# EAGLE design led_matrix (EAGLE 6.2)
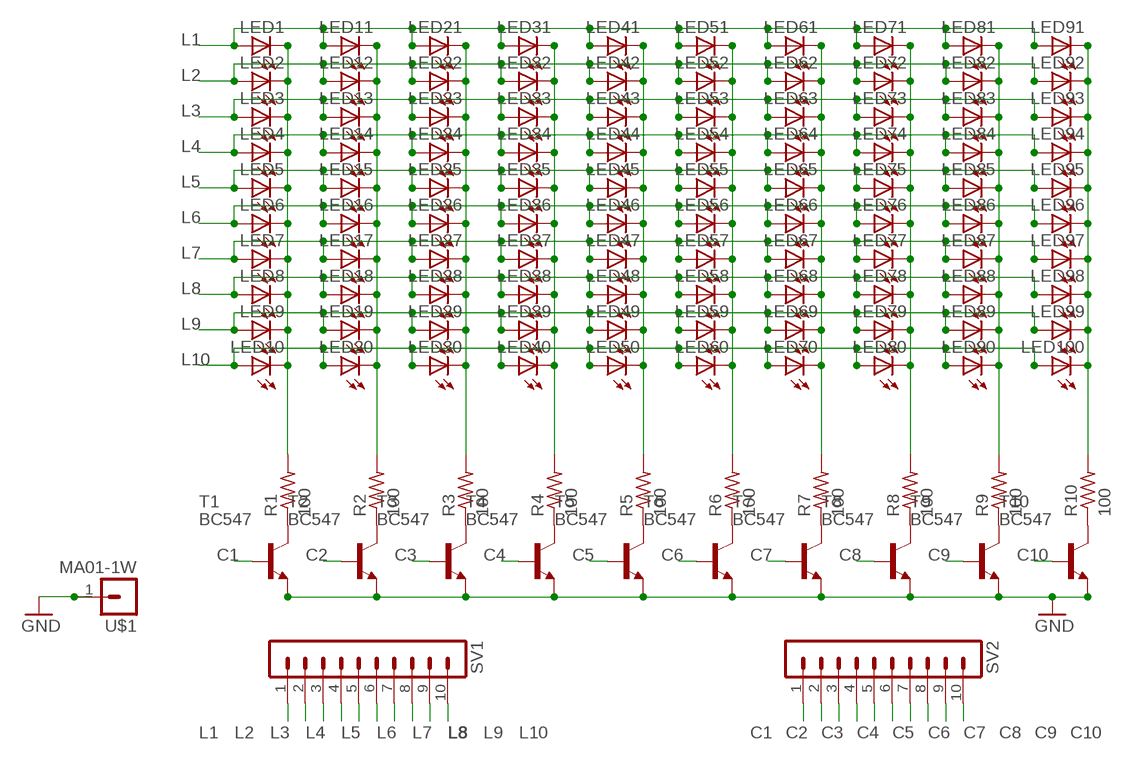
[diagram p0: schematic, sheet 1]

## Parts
LED1  LED5MM  [LED5MM]
LED2  LED5MM  [LED5MM]
LED3  LED5MM  [LED5MM]
LED4  LED5MM  [LED5MM]
LED5  LED5MM  [LED5MM]
LED6  LED5MM  [LED5MM]
LED7  LED5MM  [LED5MM]
LED8  LED5MM  [LED5MM]
LED9  LED5MM  [LED5MM]
LED10  LED5MM  [LED5MM]
LED11  LED5MM  [LED5MM]
LED12  LED5MM  [LED5MM]
LED13  LED5MM  [LED5MM]
LED14  LED5MM  [LED5MM]
LED15  LED5MM  [LED5MM]
LED16  LED5MM  [LED5MM]
LED17  LED5MM  [LED5MM]
LED18  LED5MM  [LED5MM]
LED19  LED5MM  [LED5MM]
LED20  LED5MM  [LED5MM]
LED21  LED5MM  [LED5MM]
LED22  LED5MM  [LED5MM]
LED23  LED5MM  [LED5MM]
LED24  LED5MM  [LED5MM]
LED25  LED5MM  [LED5MM]
LED26  LED5MM  [LED5MM]
LED27  LED5MM  [LED5MM]
LED28  LED5MM  [LED5MM]
LED29  LED5MM  [LED5MM]
LED30  LED5MM  [LED5MM]
LED31  LED5MM  [LED5MM]
LED32  LED5MM  [LED5MM]
LED33  LED5MM  [LED5MM]
LED34  LED5MM  [LED5MM]
LED35  LED5MM  [LED5MM]
LED36  LED5MM  [LED5MM]
LED37  LED5MM  [LED5MM]
LED38  LED5MM  [LED5MM]
LED39  LED5MM  [LED5MM]
LED40  LED5MM  [LED5MM]
LED41  LED5MM  [LED5MM]
LED42  LED5MM  [LED5MM]
LED43  LED5MM  [LED5MM]
LED44  LED5MM  [LED5MM]
LED45  LED5MM  [LED5MM]
LED46  LED5MM  [LED5MM]
LED47  LED5MM  [LED5MM]
LED48  LED5MM  [LED5MM]
LED49  LED5MM  [LED5MM]
LED50  LED5MM  [LED5MM]
LED51  LED5MM  [LED5MM]
LED52  LED5MM  [LED5MM]
LED53  LED5MM  [LED5MM]
LED54  LED5MM  [LED5MM]
LED55  LED5MM  [LED5MM]
LED56  LED5MM  [LED5MM]
LED57  LED5MM  [LED5MM]
LED58  LED5MM  [LED5MM]
LED59  LED5MM  [LED5MM]
LED60  LED5MM  [LED5MM]
LED61  LED5MM  [LED5MM]
LED62  LED5MM  [LED5MM]
LED63  LED5MM  [LED5MM]
LED64  LED5MM  [LED5MM]
LED65  LED5MM  [LED5MM]
LED66  LED5MM  [LED5MM]
LED67  LED5MM  [LED5MM]
LED68  LED5MM  [LED5MM]
LED69  LED5MM  [LED5MM]
LED70  LED5MM  [LED5MM]
LED71  LED5MM  [LED5MM]
LED72  LED5MM  [LED5MM]
LED73  LED5MM  [LED5MM]
LED74  LED5MM  [LED5MM]
LED75  LED5MM  [LED5MM]
LED76  LED5MM  [LED5MM]
LED77  LED5MM  [LED5MM]
LED78  LED5MM  [LED5MM]
LED79  LED5MM  [LED5MM]
LED80  LED5MM  [LED5MM]
LED81  LED5MM  [LED5MM]
LED82  LED5MM  [LED5MM]
LED83  LED5MM  [LED5MM]
LED84  LED5MM  [LED5MM]
LED85  LED5MM  [LED5MM]
LED86  LED5MM  [LED5MM]
LED87  LED5MM  [LED5MM]
LED88  LED5MM  [LED5MM]
LED89  LED5MM  [LED5MM]
LED90  LED5MM  [LED5MM]
LED91  LED5MM  [LED5MM]
LED92  LED5MM  [LED5MM]
LED93  LED5MM  [LED5MM]
LED94  LED5MM  [LED5MM]
LED95  LED5MM  [LED5MM]
LED96  LED5MM  [LED5MM]
LED97  LED5MM  [LED5MM]
LED98  LED5MM  [LED5MM]
LED99  LED5MM  [LED5MM]
LED100  LED5MM  [LED5MM]
R1  100  R-US_0207/10  [0207/10]
R2  100  R-US_0207/10  [0207/10]
R3  100  R-US_0207/10  [0207/10]
R4  100  R-US_0207/10  [0207/10]
R5  100  R-US_0207/10  [0207/10]
R6  100  R-US_0207/10  [0207/10]
R7  100  R-US_0207/10  [0207/10]
R8  100  R-US_0207/10  [0207/10]
R9  100  R-US_0207/10  [0207/10]
R10  100  R-US_0207/10  [0207/10]
SV1  MA10-1W  [MA10-1W]
SV2  MA10-1W  [MA10-1W]
T1  BC547  BC618  [TO92-EBC]
T2  BC547  BC618  [TO92-EBC]
T3  BC547  BC618  [TO92-EBC]
T4  BC547  BC618  [TO92-EBC]
T5  BC547  BC618  [TO92-EBC]
T6  BC547  BC618  [TO92-EBC]
T7  BC547  BC618  [TO92-EBC]
T8  BC547  BC618  [TO92-EBC]
T9  BC547  BC618  [TO92-EBC]
T10  BC547  BC618  [TO92-EBC]
U$1  MA01-1W  [MA01-1W]

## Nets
C1: SV2.1 T1.B
C2: SV2.2 T2.B
C3: SV2.3 T3.B
C4: SV2.4 T4.B
C5: SV2.5 T5.B
C6: SV2.6 T6.B
C7: SV2.7 T7.B
C8: SV2.8 T8.B
C9: SV2.9 T9.B
C10: SV2.10 T10.B
GND: T1.E T2.E T3.E T4.E T5.E T6.E T7.E T8.E T9.E T10.E U$1.1
L1: LED1.A LED11.A LED21.A LED31.A LED41.A LED51.A LED61.A LED71.A LED81.A LED91.A SV1.1
L2: LED2.A LED12.A LED22.A LED32.A LED42.A LED52.A LED62.A LED72.A LED82.A LED92.A SV1.2
L3: LED3.A LED13.A LED23.A LED33.A LED43.A LED53.A LED63.A LED73.A LED83.A LED93.A SV1.3
L4: LED4.A LED14.A LED24.A LED34.A LED44.A LED54.A LED64.A LED74.A LED84.A LED94.A SV1.4
L5: LED5.A LED15.A LED25.A LED35.A LED45.A LED55.A LED65.A LED75.A LED85.A LED95.A SV1.5
L6: LED6.A LED16.A LED26.A LED36.A LED46.A LED56.A LED66.A LED76.A LED86.A LED96.A SV1.6
L7: LED7.A LED17.A LED27.A LED37.A LED47.A LED57.A LED67.A LED77.A LED87.A LED97.A SV1.7
L8: LED8.A LED18.A LED28.A LED38.A LED48.A LED58.A LED68.A LED78.A LED88.A LED98.A SV1.8
L9: LED9.A LED19.A LED29.A LED39.A LED49.A LED59.A LED69.A LED79.A LED89.A LED99.A SV1.9
L10: LED10.A LED20.A LED30.A LED40.A LED50.A LED60.A LED70.A LED80.A LED90.A LED100.A SV1.10
N$1: R1.1 T1.C
N$2: R2.1 T2.C
N$3: R3.1 T3.C
N$4: R4.1 T4.C
N$5: R5.1 T5.C
N$6: R6.1 T6.C
N$7: R7.1 T7.C
N$8: R8.1 T8.C
N$9: R9.1 T9.C
N$10: R10.1 T10.C
N$11: LED1.K(C) LED2.K(C) LED3.K(C) LED4.K(C) LED5.K(C) LED6.K(C) LED7.K(C) LED8.K(C) LED9.K(C) LED10.K(C) R1.2
N$12: LED11.K(C) LED12.K(C) LED13.K(C) LED14.K(C) LED15.K(C) LED16.K(C) LED17.K(C) LED18.K(C) LED19.K(C) LED20.K(C) R2.2
N$13: LED21.K(C) LED22.K(C) LED23.K(C) LED24.K(C) LED25.K(C) LED26.K(C) LED27.K(C) LED28.K(C) LED29.K(C) LED30.K(C) R3.2
N$14: LED31.K(C) LED32.K(C) LED33.K(C) LED34.K(C) LED35.K(C) LED36.K(C) LED37.K(C) LED38.K(C) LED39.K(C) LED40.K(C) R4.2
N$15: LED41.K(C) LED42.K(C) LED43.K(C) LED44.K(C) LED45.K(C) LED46.K(C) LED47.K(C) LED48.K(C) LED49.K(C) LED50.K(C) R5.2
N$16: LED51.K(C) LED52.K(C) LED53.K(C) LED54.K(C) LED55.K(C) LED56.K(C) LED57.K(C) LED58.K(C) LED59.K(C) LED60.K(C) R6.2
N$17: LED61.K(C) LED62.K(C) LED63.K(C) LED64.K(C) LED65.K(C) LED66.K(C) LED67.K(C) LED68.K(C) LED69.K(C) LED70.K(C) R7.2
N$18: LED71.K(C) LED72.K(C) LED73.K(C) LED74.K(C) LED75.K(C) LED76.K(C) LED77.K(C) LED78.K(C) LED79.K(C) LED80.K(C) R8.2
N$19: LED81.K(C) LED82.K(C) LED83.K(C) LED84.K(C) LED85.K(C) LED86.K(C) LED87.K(C) LED88.K(C) LED89.K(C) LED90.K(C) R9.2
N$20: LED91.K(C) LED92.K(C) LED93.K(C) LED94.K(C) LED95.K(C) LED96.K(C) LED97.K(C) LED98.K(C) LED99.K(C) LED100.K(C) R10.2

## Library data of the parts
LED1-LED100 = SparkFun-LED:LED: LEDs
R1-R10 = rcl:R-US_: RESISTOR, American symbol
SV1 SV2 = con-lstb:MA10-1W: PIN HEADER; OC_FARNELL: unknown; OC_NEWARK: unknown
T1-T10 = transistor-npn:BC618*: NPN Transistor
U$1 = con-lstb:MA01-1W

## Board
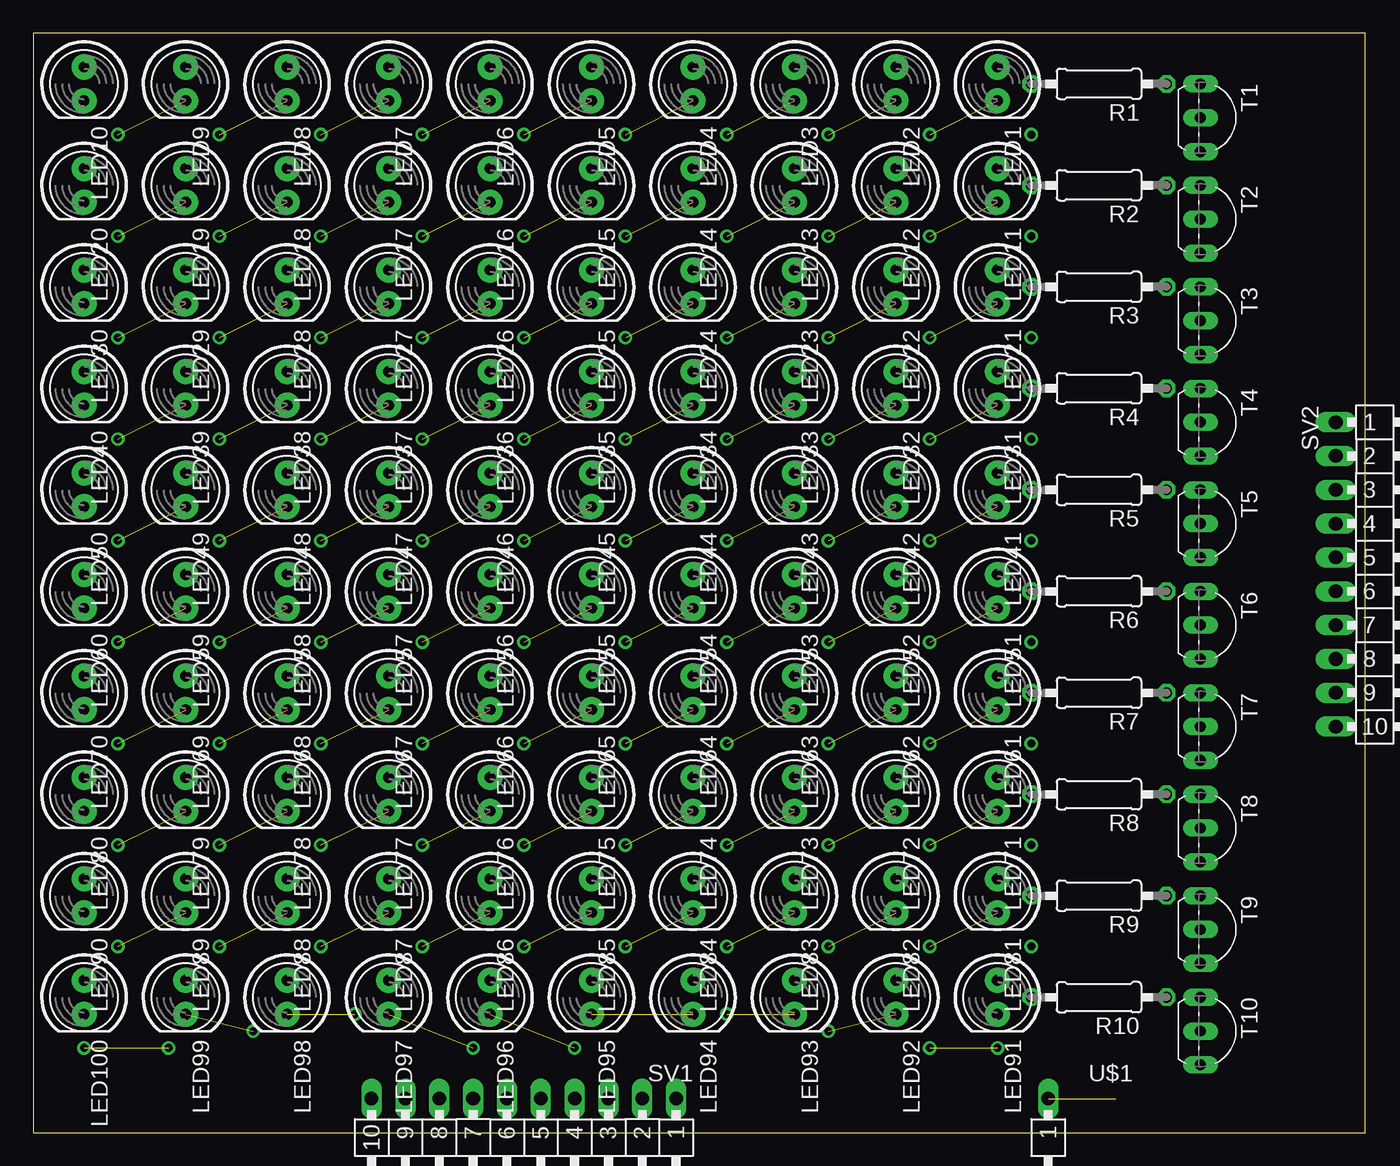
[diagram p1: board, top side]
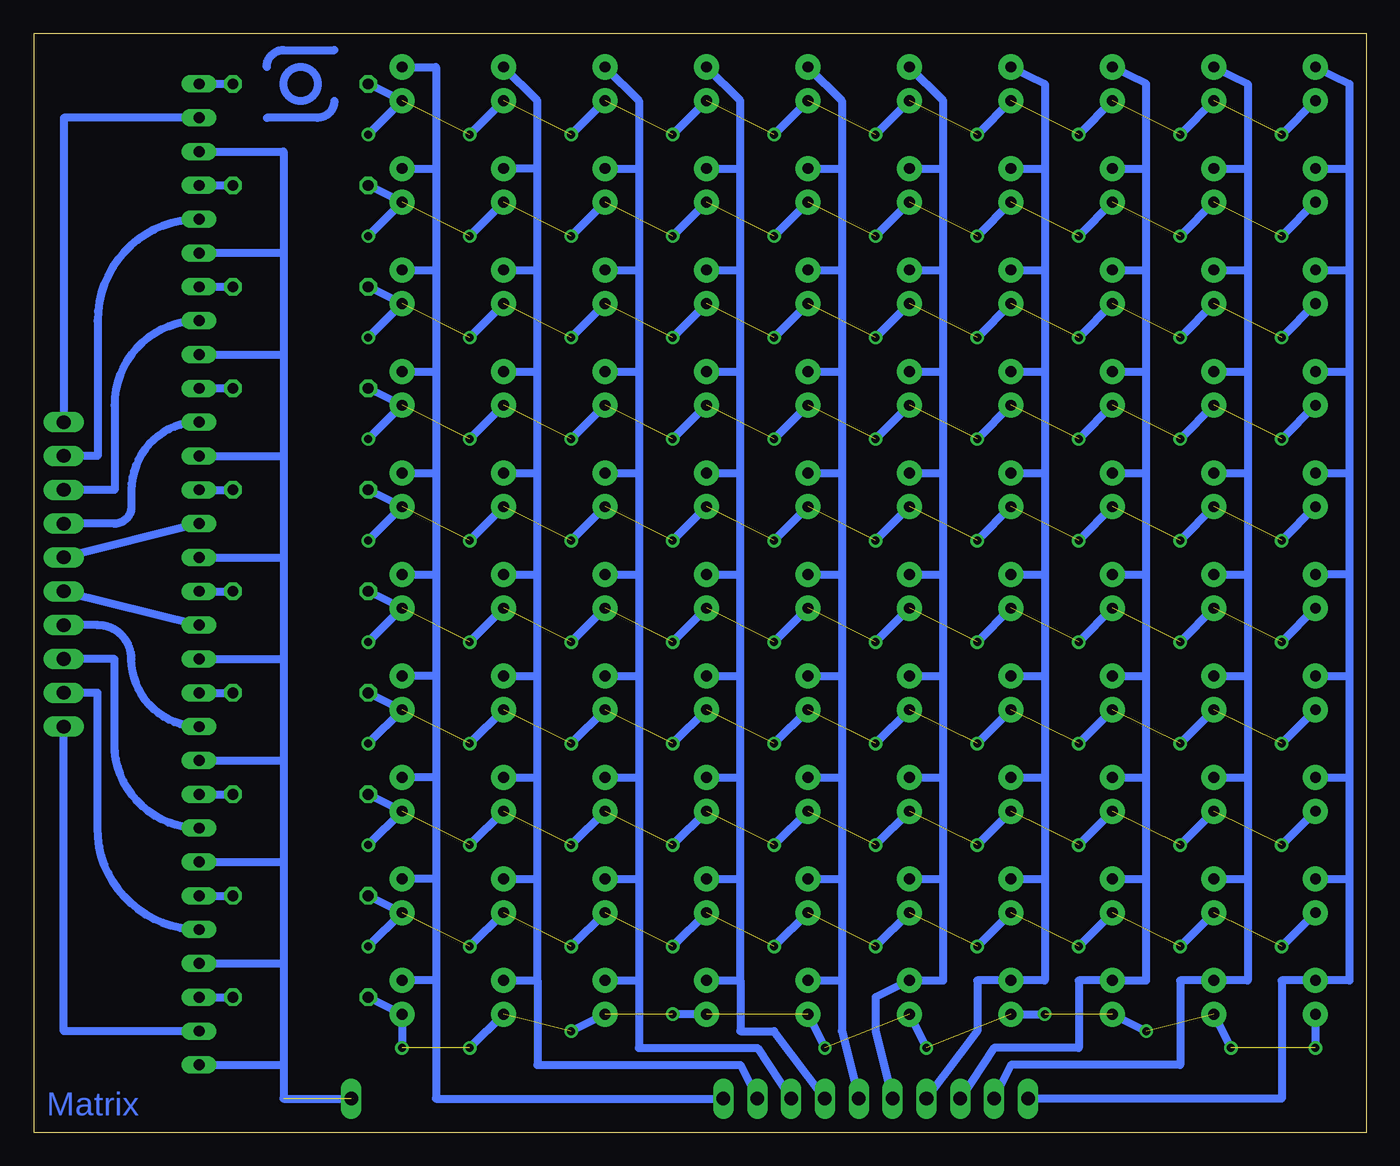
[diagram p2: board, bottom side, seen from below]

Size 100 x 82.54 mm. Coordinates in mm from the lower left corner, seen from the top.
Outline: 0,0 100,0 100,82.54 0,82.54 0,0
Copper layers (1*16): Top 0.035mm / dielectric 1.5mm / Bottom 0.035mm
Design rules: minimum track width 0.5mm, minimum drill 0.6mm, track to track 0.5mm, track to pad 0.5mm, pad to pad 0.5mm, via to via 0.5mm, smd to smd 8mil, copper to edge 0.4mm, drill to drill 8mil, minimum pad ring 10mil, minimum via ring 8mil, stop-mask expansion 4mil, vias tented up to drill 0mil, thermal gap 10mil

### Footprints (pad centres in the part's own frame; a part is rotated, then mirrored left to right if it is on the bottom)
LED5MM = drill 0.813 pad 1.88: A -1.27,0; K 1.27,0
0207/10 = drill 0.813 octagon: 1 -5.08,0; 2 5.08,0
MA10-1W = drill 1.016 long: 1 -11.43,0; 2 -8.89,0; 3 -6.35,0; 4 -3.81,0; 5 -1.27,0; 6 1.27,0; 7 3.81,0; 8 6.35,0; 9 8.89,0; 10 11.43,0
TO92-EBC = drill 0.813 long: B 0,-1.27; C -2.54,-1.27; E 2.54,-1.27
MA01-1W = drill 1.016 long: 1 6.35,2.54

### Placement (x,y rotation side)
LED1  72.39,78.74 270 top
LED2  64.77,78.74 270 top
LED3  57.15,78.74 270 top
LED4  49.53,78.74 270 top
LED5  41.91,78.74 270 top
LED6  34.29,78.74 270 top
LED7  26.67,78.74 270 top
LED8  19.05,78.74 270 top
LED9  11.43,78.74 270 top
LED10  3.81,78.74 270 top
LED11  72.39,71.12 270 top
LED12  64.77,71.12 270 top
LED13  57.15,71.12 270 top
LED14  49.53,71.12 270 top
LED15  41.91,71.12 270 top
LED16  34.29,71.12 270 top
LED17  26.67,71.12 270 top
LED18  19.05,71.12 270 top
LED19  11.43,71.12 270 top
LED20  3.81,71.12 270 top
LED21  72.39,63.5 270 top
LED22  64.77,63.5 270 top
LED23  57.15,63.5 270 top
LED24  49.53,63.5 270 top
LED25  41.91,63.5 270 top
LED26  34.29,63.5 270 top
LED27  26.67,63.5 270 top
LED28  19.05,63.5 270 top
LED29  11.43,63.5 270 top
LED30  3.81,63.5 270 top
LED31  72.39,55.88 270 top
LED32  64.77,55.88 270 top
LED33  57.15,55.88 270 top
LED34  49.53,55.88 270 top
LED35  41.91,55.88 270 top
LED36  34.29,55.88 270 top
LED37  26.67,55.88 270 top
LED38  19.05,55.88 270 top
LED39  11.43,55.88 270 top
LED40  3.81,55.88 270 top
LED41  72.39,48.26 270 top
LED42  64.77,48.26 270 top
LED43  57.15,48.26 270 top
LED44  49.53,48.26 270 top
LED45  41.91,48.26 270 top
LED46  34.29,48.26 270 top
LED47  26.67,48.26 270 top
LED48  19.05,48.26 270 top
LED49  11.43,48.26 270 top
LED50  3.81,48.26 270 top
LED51  72.39,40.64 270 top
LED52  64.77,40.64 270 top
LED53  57.15,40.64 270 top
LED54  49.53,40.64 270 top
LED55  41.91,40.64 270 top
LED56  34.29,40.64 270 top
LED57  26.67,40.64 270 top
LED58  19.05,40.64 270 top
LED59  11.43,40.64 270 top
LED60  3.81,40.64 270 top
LED61  72.39,33.02 270 top
LED62  64.77,33.02 270 top
LED63  57.15,33.02 270 top
LED64  49.53,33.02 270 top
LED65  41.91,33.02 270 top
LED66  34.29,33.02 270 top
LED67  26.67,33.02 270 top
LED68  19.05,33.02 270 top
LED69  11.43,33.02 270 top
LED70  3.81,33.02 270 top
LED71  72.39,25.4 270 top
LED72  64.77,25.4 270 top
LED73  57.15,25.4 270 top
LED74  49.53,25.4 270 top
LED75  41.91,25.4 270 top
LED76  34.29,25.4 270 top
LED77  26.67,25.4 270 top
LED78  19.05,25.4 270 top
LED79  11.43,25.4 270 top
LED80  3.81,25.4 270 top
LED81  72.39,17.78 270 top
LED82  64.77,17.78 270 top
LED83  57.15,17.78 270 top
LED84  49.53,17.78 270 top
LED85  41.91,17.78 270 top
LED86  34.29,17.78 270 top
LED87  26.67,17.78 270 top
LED88  19.05,17.78 270 top
LED89  11.43,17.78 270 top
LED90  3.81,17.78 270 top
LED91  72.39,10.16 270 top
LED92  64.77,10.16 270 top
LED93  57.15,10.16 270 top
LED94  49.53,10.16 270 top
LED95  41.91,10.16 270 top
LED96  34.29,10.16 270 top
LED97  26.67,10.16 270 top
LED98  19.05,10.16 270 top
LED99  11.43,10.16 270 top
LED100  3.81,10.16 270 top
R1  80.01,78.74 180 top
R2  80.01,71.12 180 top
R3  80.01,63.5 180 top
R4  80.01,55.88 180 top
R5  80.01,48.26 180 top
R6  80.01,40.64 180 top
R7  80.01,33.02 180 top
R8  80.01,25.4 180 top
R9  80.01,17.78 180 top
R10  80.01,10.16 180 top
SV1  36.83,2.54 180 top
SV2  97.79,41.91 270 top
T1  88.9,76.2 270 top
T2  88.9,68.58 270 top
T3  88.9,60.96 270 top
T4  88.9,53.34 270 top
T5  88.9,45.72 270 top
T6  88.9,38.1 270 top
T7  88.9,30.48 270 top
T8  88.9,22.86 270 top
T9  88.9,15.24 270 top
T10  88.9,7.62 270 top
U$1  82.55,5.08 180 top

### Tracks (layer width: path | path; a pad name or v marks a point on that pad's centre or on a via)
C1
  Bottom 0.6: T1.B 97.79,76.2 SV2.1
C2
  Bottom 0.6: T2.B arc-90 95.25,60.96 95.25,50.8 SV2.2
C3
  Bottom 0.6: T3.B arc-90 93.98,54.61 93.98,48.26 SV2.3
C4
  Bottom 0.6: T4.B arc-90 92.71,48.26 92.71,46.99 arc90 93.98,45.72 SV2.4
C5
  Bottom 0.6: T5.B SV2.5
C6
  Bottom 0.6: SV2.6 T6.B
C7
  Bottom 0.6: T7.B arc90 92.71,35.56 arc-90 95.25,38.1 SV2.7
C8
  Bottom 0.6: T8.B arc90 93.98,29.21 93.98,35.56 SV2.8
C9
  Bottom 0.6: T9.B arc90 95.25,22.86 95.25,33.02 SV2.9
C10
  Bottom 0.6: T10.B 97.79,7.62 SV2.10
GND  (1 unrouted)
  Bottom 0.6: T1.E 81.28,73.66 81.28,66.04 | 81.28,66.04 81.28,58.42 | 81.28,58.42 81.28,50.8 | 81.28,50.8 81.28,43.18 | 81.28,43.18 81.28,35.56 | 81.28,35.56 81.28,27.94 | 81.28,27.94 81.28,20.32 | 81.28,20.32 81.28,12.7 | 81.28,12.7 81.28,5.08 | 81.28,5.08 81.28,2.54 U$1.1 | T10.E 81.28,5.08 | 81.28,66.04 T2.E | T3.E 81.28,58.42 | T4.E 81.28,50.8 | T5.E 81.28,43.18 | T6.E 81.28,35.56 | T7.E 81.28,27.94 | T8.E 81.28,20.32 | T9.E 81.28,12.7
L1
  Bottom 0.6: LED1.A 69.85,80.01 69.85,72.39 | 69.85,72.39 69.85,64.77 | 69.85,64.77 69.85,57.15 | 69.85,57.15 69.85,49.53 | 69.85,49.53 69.85,41.91 | 69.85,41.91 69.85,34.29 | 69.85,34.29 69.85,26.67 | 69.85,26.67 69.85,19.05 | 69.85,19.05 69.85,11.43 | 69.85,11.43 69.85,2.54 SV1.1 | 69.85,11.43 LED91.A | 69.85,19.05 LED81.A | 69.85,26.67 LED71.A | 69.85,34.29 LED61.A | LED51.A 69.85,41.91 | LED41.A 69.85,49.53 | LED31.A 69.85,57.15 | LED21.A 69.85,64.77 | LED11.A 69.85,72.39
L2
  Bottom 0.6: LED92.A 62.23,11.43 | 62.23,11.43 62.23,5.08 46.99,5.08 SV1.2 | 62.23,11.43 62.23,19.05 | 62.23,19.05 62.23,26.67 | 62.23,26.67 62.23,34.29 | 62.23,34.29 62.23,41.91 | 62.23,41.91 62.23,49.53 | 62.23,49.53 62.23,57.15 | 62.23,57.15 62.23,64.77 | 62.23,64.77 62.23,72.39 | 62.23,72.39 62.23,77.47 LED2.A | LED82.A 62.23,19.05 | LED72.A 62.23,26.67 | LED62.A 62.23,34.29 | LED52.A 62.23,41.91 | LED42.A 62.23,49.53 | LED32.A 62.23,57.15 | LED22.A 62.23,64.77 | 62.23,72.39 LED12.A
L3
  Bottom 0.6: LED93.A 54.61,11.43 | 54.61,11.43 54.61,6.35 45.72,6.35 SV1.3 | LED3.A 54.61,77.47 54.61,72.39 | 54.61,72.39 54.61,64.77 | 54.61,64.77 54.61,57.15 | 54.61,57.15 54.61,49.53 | 54.61,49.53 54.61,41.91 | 54.61,41.91 54.61,34.29 | 54.61,34.29 54.61,26.67 | 54.61,26.67 54.61,19.05 | 54.61,19.05 54.61,11.43 | LED13.A 54.61,72.39 | LED23.A 54.61,64.77 | LED33.A 54.61,57.15 | LED43.A 54.61,49.53 | LED53.A 54.61,41.91 | LED63.A 54.61,34.29 | LED73.A 54.61,26.67 | LED83.A 54.61,19.05
L4
  Bottom 0.6: LED94.A 46.99,11.43 | 46.99,11.43 46.99,7.62 44.45,7.62 SV1.4 | 46.99,11.43 46.99,19.05 | 46.99,19.05 46.99,26.67 | 46.99,26.67 46.99,34.29 | 46.99,34.29 46.99,41.91 | 46.99,41.91 46.99,49.53 | 46.99,49.53 46.99,57.15 | 46.99,57.15 46.99,64.77 | 46.99,64.77 46.99,72.39 | 46.99,72.39 46.99,77.47 LED4.A | LED84.A 46.99,19.05 | LED74.A 46.99,26.67 | LED64.A 46.99,34.29 | LED54.A 46.99,41.91 | LED44.A 46.99,49.53 | LED34.A 46.99,57.15 | LED24.A 46.99,64.77 | LED14.A 46.99,72.39
L5
  Bottom 0.6: LED95.A 39.37,11.43 | 39.37,11.43 39.37,7.62 SV1.5 | LED5.A 39.37,77.47 39.37,72.39 | 39.37,72.39 39.37,64.77 | 39.37,64.77 39.37,57.15 | 39.37,57.15 39.37,49.53 | 39.37,49.53 39.37,41.91 | 39.37,41.91 39.37,34.29 | 39.37,34.29 39.37,26.67 | 39.37,26.67 39.37,19.05 | 39.37,19.05 39.37,11.43 | LED25.A 39.37,64.77 | LED15.A 39.37,72.39 | LED35.A 39.37,57.15 | LED45.A 39.37,49.53 | LED55.A 39.37,41.91 | LED65.A 39.37,34.29 | LED75.A 39.37,26.67 | LED85.A 39.37,19.05
L6
  Bottom 0.6: SV1.6 36.83,7.62 36.83,10.16 LED96.A 31.75,11.43 31.75,19.05 | 31.75,19.05 31.75,26.67 | 31.75,26.67 31.75,34.29 | 31.75,34.29 31.75,41.91 | 31.75,41.91 31.75,49.53 | 31.75,49.53 31.75,57.15 | 31.75,57.15 31.75,64.77 | 31.75,64.77 31.75,72.39 | 31.75,72.39 31.75,77.47 LED6.A | LED86.A 31.75,19.05 | LED76.A 31.75,26.67 | LED66.A 31.75,34.29 | LED56.A 31.75,41.91 | LED46.A 31.75,49.53 | LED36.A 31.75,57.15 | LED26.A 31.75,64.77 | LED16.A 31.75,72.39
L7
  Bottom 0.6: SV1.7 29.21,7.62 29.21,11.43 LED97.A 24.13,11.43 24.13,19.05 | LED7.A 24.13,78.74 24.13,72.39 | 24.13,72.39 24.13,64.77 | 24.13,64.77 24.13,57.15 | 24.13,57.15 24.13,49.53 | 24.13,49.53 24.13,41.91 | 24.13,41.91 24.13,34.29 | 24.13,34.29 24.13,26.67 | 24.13,26.67 24.13,19.05 | LED87.A 24.13,19.05 | LED77.A 24.13,26.67 | LED67.A 24.13,34.29 | LED57.A 24.13,41.91 | LED47.A 24.13,49.53 | LED37.A 24.13,57.15 | LED27.A 24.13,64.77 | LED17.A 24.13,72.39
L8
  Bottom 0.6: SV1.8 27.94,6.35 21.59,6.35 21.59,11.43 LED98.A 16.51,11.43 16.51,19.05 | 16.51,19.05 16.51,26.67 | 16.51,26.67 16.51,34.29 | 16.51,34.29 16.51,41.91 | 16.51,41.91 16.51,49.53 | 16.51,49.53 16.51,57.15 | 16.51,57.15 16.51,64.77 | 16.51,64.77 16.51,72.39 | 16.51,72.39 16.51,78.74 LED8.A | LED18.A 16.51,72.39 | LED28.A 16.51,64.77 | LED38.A 16.51,57.15 | LED48.A 16.51,49.53 | LED58.A 16.51,41.91 | LED68.A 16.51,34.29 | LED78.A 16.51,26.67 | LED88.A 16.51,19.05
L9
  Bottom 0.6: SV1.9 26.67,5.08 13.97,5.08 13.97,11.43 LED99.A 8.89,11.43 8.89,19.05 | LED9.A 8.89,78.74 8.89,72.39 | 8.89,72.39 8.89,64.77 | 8.89,64.77 8.89,57.15 | 8.89,57.15 8.89,49.53 | 8.89,49.53 8.89,41.91 | 8.89,41.91 8.89,34.29 | 8.89,34.29 8.89,26.67 | 8.89,26.67 8.89,19.05 | LED19.A 8.89,72.39 | LED29.A 8.89,64.77 | LED89.A 8.89,19.05 | LED79.A 8.89,26.67 | LED69.A 8.89,34.29 | LED59.A 8.89,41.91 | LED49.A 8.89,49.53 | LED39.A 8.89,57.15
L10
  Bottom 0.6: SV1.10 6.35,2.54 6.35,11.43 LED100.A 1.27,11.43 1.27,19.05 | LED10.A 1.27,78.74 1.27,72.39 | 1.27,72.39 1.27,64.77 | 1.27,64.77 1.27,57.15 | 1.27,57.15 1.27,49.53 | 1.27,49.53 1.27,41.91 | 1.27,41.91 1.27,34.29 | 1.27,34.29 1.27,26.67 | 1.27,26.67 1.27,19.05 | LED20.A 1.27,72.39 | LED30.A 1.27,64.77 | LED40.A 1.27,57.15 | LED50.A 1.27,49.53 | 1.27,41.91 LED60.A | LED70.A 1.27,34.29 | LED80.A 1.27,26.67 | LED90.A 1.27,19.05
N$1
  Bottom 0.6: T1.C R1.1
N$2
  Bottom 0.6: T2.C R2.1
N$3
  Bottom 0.6: T3.C R3.1
N$4
  Bottom 0.6: R4.1 T4.C
N$5
  Bottom 0.6: T5.C R5.1
N$6
  Bottom 0.6: T6.C R6.1
N$7
  Bottom 0.6: T7.C R7.1
N$8
  Bottom 0.6: T8.C R8.1
N$9
  Bottom 0.6: T9.C R9.1
N$10
  Bottom 0.6: T10.C R10.1
N$11  (via drill 0.6)  (9 unrouted)
  Bottom 0.6: v67.31,74.93 LED2.K | LED3.K v59.69,74.93 | LED10.K v6.35,74.93 | LED9.K v13.97,74.93 | LED8.K v21.59,74.93 | LED7.K v29.21,74.93 | LED6.K v36.83,74.93 | LED5.K v44.45,74.93 | LED4.K v52.07,74.93 | v74.93,74.93 LED1.K R1.2
N$12  (via drill 0.6)  (9 unrouted)
  Bottom 0.6: LED12.K v67.31,67.31 | LED13.K v59.69,67.31 | v52.07,67.31 LED14.K | LED20.K v6.35,67.31 | LED19.K v13.97,67.31 | LED18.K v21.59,67.31 | LED17.K v29.21,67.31 | LED16.K v36.83,67.31 | LED15.K v44.45,67.31 | v74.93,67.31 LED11.K R2.2
N$13  (via drill 0.6)  (9 unrouted)
  Bottom 0.6: LED22.K v67.31,59.69 | LED30.K v6.35,59.69 | LED29.K v13.97,59.69 | LED28.K v21.59,59.69 | LED23.K v59.69,59.69 | LED24.K v52.07,59.69 | LED25.K v44.45,59.69 | LED26.K v36.83,59.69 | LED27.K v29.21,59.69 | v74.93,59.69 LED21.K R3.2
N$14  (via drill 0.6)  (9 unrouted)
  Bottom 0.6: LED32.K v67.31,52.07 | LED33.K v59.69,52.07 | LED34.K v52.07,52.07 | LED35.K v44.45,52.07 | LED36.K v36.83,52.07 | LED37.K v29.21,52.07 | LED38.K v21.59,52.07 | LED39.K v13.97,52.07 | LED40.K v6.35,52.07 | v74.93,52.07 LED31.K R4.2
N$15  (via drill 0.6)  (9 unrouted)
  Bottom 0.6: LED42.K v67.31,44.45 | LED50.K v6.35,44.45 | LED49.K v13.97,44.45 | LED48.K v21.59,44.45 | LED47.K v29.21,44.45 | LED46.K v36.83,44.45 | LED45.K v44.45,44.45 | LED44.K v52.07,44.45 | LED43.K v59.69,44.45 | v74.93,44.45 LED41.K R5.2
N$16  (via drill 0.6)  (9 unrouted)
  Bottom 0.6: LED52.K v67.31,36.83 | LED53.K v59.69,36.83 | LED54.K v52.07,36.83 | LED55.K v44.45,36.83 | LED56.K v36.83,36.83 | LED57.K v29.21,36.83 | LED58.K v21.59,36.83 | LED59.K v13.97,36.83 | LED60.K v6.35,36.83 | v74.93,36.83 LED51.K R6.2
N$17  (via drill 0.6)  (9 unrouted)
  Bottom 0.6: LED62.K v67.31,29.21 | LED63.K v59.69,29.21 | LED64.K v52.07,29.21 | LED65.K v44.45,29.21 | LED66.K v36.83,29.21 | LED67.K v29.21,29.21 | LED68.K v21.59,29.21 | LED69.K v13.97,29.21 | LED70.K v6.35,29.21 | v74.93,29.21 LED61.K R7.2
N$18  (via drill 0.6)  (9 unrouted)
  Bottom 0.6: LED72.K v67.31,21.59 | LED80.K v6.35,21.59 | LED79.K v13.97,21.59 | LED78.K v21.59,21.59 | LED77.K v29.21,21.59 | LED76.K v36.83,21.59 | LED75.K v44.45,21.59 | LED74.K v52.07,21.59 | LED73.K v59.69,21.59 | v74.93,21.59 LED71.K R8.2
N$19  (via drill 0.6)  (9 unrouted)
  Bottom 0.6: LED82.K v67.31,13.97 | LED90.K v6.35,13.97 | LED89.K v13.97,13.97 | LED88.K v21.59,13.97 | LED87.K v29.21,13.97 | LED86.K v36.83,13.97 | LED85.K v44.45,13.97 | LED84.K v52.07,13.97 | LED83.K v59.69,13.97 | v74.93,13.97 LED81.K R9.2
N$20  (via drill 0.6)  (9 unrouted)
  Bottom 0.6: LED92.K v67.31,6.35 | LED93.K v59.69,7.62 | LED94.K v52.07,8.89 | LED95.K v40.64,6.35 | LED96.K v33.02,6.35 | LED97.K v24.13,8.89 | LED98.K v16.51,7.62 | LED99.K v10.16,6.35 | LED100.K v3.81,6.35 | v72.39,6.35 LED91.K R10.2
N$21
  Bottom 0.6: 82.55,80.01 arc90 81.28,81.28 77.47,81.28
N$22
  Bottom 0.6: 77.47,77.47 arc90 78.74,76.2 82.55,76.2
(copper drawn outside any net)
  shapes: Bottom circle x1

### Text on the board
Bottom: Matrix

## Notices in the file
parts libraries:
SparkFun-LED: Licensing: CC v3.0 Share-Alike You are welcome to use this library for commercial purposes.
